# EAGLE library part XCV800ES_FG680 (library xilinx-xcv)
xcv800es_fg680 edit this description Auto generated by make-symbol-device-package-bsdl.ulp Rev. 26 Source: xcv800es_fg680.bsd
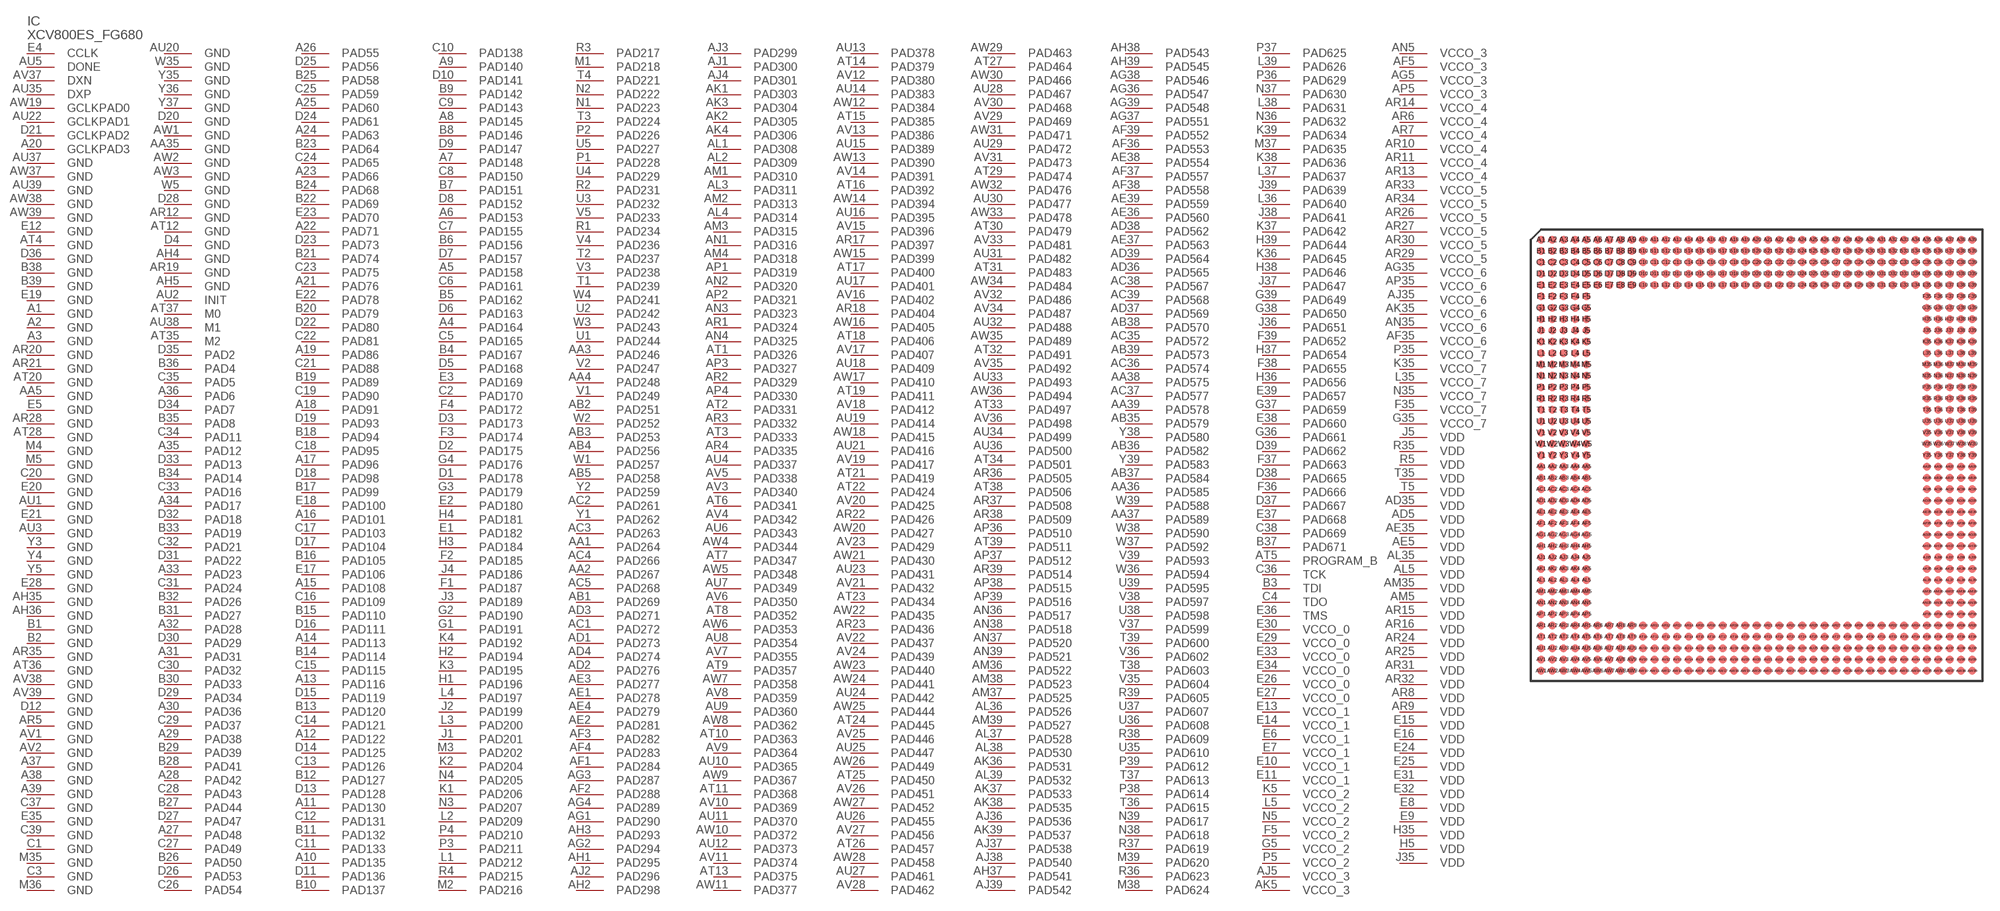
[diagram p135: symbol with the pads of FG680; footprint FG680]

Designator prefix IC

## XCV800ES_FG680 (OC_FARNELL: unknown; OC_NEWARK: unknown)  [FG680]
A1  GND  pwr
A2  GND  pwr
A3  GND  pwr
A4  PAD164
A5  PAD158
A6  PAD153
A7  PAD148
A8  PAD145
A9  PAD140
A10  PAD135
A11  PAD130
A12  PAD122
A13  PAD116
A14  PAD113
A15  PAD108
A16  PAD101
A17  PAD96
A18  PAD91
A19  PAD86
A20  GCLKPAD3  in
A21  PAD76
A22  PAD71
A23  PAD66
A24  PAD63
A25  PAD60
A26  PAD55
A27  PAD48
A28  PAD42
A29  PAD38
A30  PAD36
A31  PAD31
A32  PAD28
A33  PAD23
A34  PAD17
A35  PAD12
A36  PAD6
A37  GND  pwr
A38  GND  pwr
A39  GND  pwr
AA1  PAD264
AA2  PAD267
AA3  PAD246
AA4  PAD248
AA5  GND  pwr
AA35  GND  pwr
AA36  PAD585
AA37  PAD589
AA38  PAD575
AA39  PAD578
AB1  PAD269
AB2  PAD251
AB3  PAD253
AB4  PAD256
AB5  PAD258
AB35  PAD579
AB36  PAD582
AB37  PAD584
AB38  PAD570
AB39  PAD573
AC1  PAD272
AC2  PAD261
AC3  PAD263
AC4  PAD266
AC5  PAD268
AC35  PAD572
AC36  PAD574
AC37  PAD577
AC38  PAD567
AC39  PAD568
AD1  PAD273
AD2  PAD276
AD3  PAD271
AD4  PAD274
AD5  VDD  pwr
AD35  VDD  pwr
AD36  PAD565
AD37  PAD569
AD38  PAD562
AD39  PAD564
AE1  PAD278
AE2  PAD281
AE3  PAD277
AE4  PAD279
AE5  VDD  pwr
AE35  VDD  pwr
AE36  PAD560
AE37  PAD563
AE38  PAD554
AE39  PAD559
AF1  PAD284
AF2  PAD288
AF3  PAD282
AF4  PAD283
AF5  VCCO_3  pwr
AF35  VCCO_6  pwr
AF36  PAD553
AF37  PAD557
AF38  PAD558
AF39  PAD552
AG1  PAD290
AG2  PAD294
AG3  PAD287
AG4  PAD289
AG5  VCCO_3  pwr
AG35  VCCO_6  pwr
AG36  PAD547
AG37  PAD551
AG38  PAD546
AG39  PAD548
AH1  PAD295
AH2  PAD298
AH3  PAD293
AH4  GND  pwr
AH5  GND  pwr
AH35  GND  pwr
AH36  GND  pwr
AH37  PAD541
AH38  PAD543
AH39  PAD545
AJ1  PAD300
AJ2  PAD296
AJ3  PAD299
AJ4  PAD301
AJ5  VCCO_3  pwr
AJ35  VCCO_6  pwr
AJ36  PAD536
AJ37  PAD538
AJ38  PAD540
AJ39  PAD542
AK1  PAD303
AK2  PAD305
AK3  PAD304
AK4  PAD306
AK5  VCCO_3  pwr
AK35  VCCO_6  pwr
AK36  PAD531
AK37  PAD533
AK38  PAD535
AK39  PAD537
AL1  PAD308
AL2  PAD309
AL3  PAD311
AL4  PAD314
AL5  VDD  pwr
AL35  VDD  pwr
AL36  PAD526
AL37  PAD528
AL38  PAD530
AL39  PAD532
AM1  PAD310
AM2  PAD313
AM3  PAD315
AM4  PAD318
AM5  VDD  pwr
AM35  VDD  pwr
AM36  PAD522
AM37  PAD525
AM38  PAD523
AM39  PAD527
AN1  PAD316
AN2  PAD320
AN3  PAD323
AN4  PAD325
AN5  VCCO_3  pwr
AN35  VCCO_6  pwr
AN36  PAD517
AN37  PAD520
AN38  PAD518
AN39  PAD521
AP1  PAD319
AP2  PAD321
AP3  PAD327
AP4  PAD330
AP5  VCCO_3  pwr
AP35  VCCO_6  pwr
AP36  PAD510
AP37  PAD512
AP38  PAD515
AP39  PAD516
AR1  PAD324
AR2  PAD329
AR3  PAD332
AR4  PAD335
AR5  GND  pwr
AR6  VCCO_4  pwr
AR7  VCCO_4  pwr
AR8  VDD  pwr
AR9  VDD  pwr
AR10  VCCO_4  pwr
AR11  VCCO_4  pwr
AR12  GND  pwr
AR13  VCCO_4  pwr
AR14  VCCO_4  pwr
AR15  VDD  pwr
AR16  VDD  pwr
AR17  PAD397
AR18  PAD404
AR19  GND  pwr
AR20  GND  pwr
AR21  GND  pwr
AR22  PAD426
AR23  PAD436
AR24  VDD  pwr
AR25  VDD  pwr
AR26  VCCO_5  pwr
AR27  VCCO_5  pwr
AR28  GND  pwr
AR29  VCCO_5  pwr
AR30  VCCO_5  pwr
AR31  VDD  pwr
AR32  VDD  pwr
AR33  VCCO_5  pwr
AR34  VCCO_5  pwr
AR35  GND  pwr
AR36  PAD505
AR37  PAD508
AR38  PAD509
AR39  PAD514
AT1  PAD326
AT2  PAD331
AT3  PAD333
AT4  GND  pwr
AT5  PROGRAM_B  in
AT6  PAD341
AT7  PAD347
AT8  PAD352
AT9  PAD357
AT10  PAD363
AT11  PAD368
AT12  GND  pwr
AT13  PAD375
AT14  PAD379
AT15  PAD385
AT16  PAD392
AT17  PAD400
AT18  PAD406
AT19  PAD411
AT20  GND  pwr
AT21  PAD419
AT22  PAD424
AT23  PAD434
AT24  PAD445
AT25  PAD450
AT26  PAD457
AT27  PAD464
AT28  GND  pwr
AT29  PAD474
AT30  PAD479
AT31  PAD483
AT32  PAD491
AT33  PAD497
AT34  PAD501
AT35  M2  in
AT36  GND  pwr
AT37  M0  in
AT38  PAD506
AT39  PAD511
AU1  GND  pwr
AU2  INIT
AU3  GND  pwr
AU4  PAD337
AU5  DONE
AU6  PAD343
AU7  PAD349
AU8  PAD354
AU9  PAD360
AU10  PAD365
AU11  PAD370
AU12  PAD373
AU13  PAD378
AU14  PAD383
AU15  PAD389
AU16  PAD395
AU17  PAD401
AU18  PAD409
AU19  PAD414
AU20  GND  pwr
AU21  PAD416
AU22  GCLKPAD1  in
AU23  PAD431
AU24  PAD442
AU25  PAD447
AU26  PAD455
AU27  PAD461
AU28  PAD467
AU29  PAD472
AU30  PAD477
AU31  PAD482
AU32  PAD488
AU33  PAD493
AU34  PAD499
AU35  DXP  pas
AU36  PAD500
AU37  GND  pwr
AU38  M1  in
AU39  GND  pwr
AV1  GND  pwr
AV2  GND  pwr
AV3  PAD340
AV4  PAD342
AV5  PAD338
AV6  PAD350
AV7  PAD355
AV8  PAD359
AV9  PAD364
AV10  PAD369
AV11  PAD374
AV12  PAD380
AV13  PAD386
AV14  PAD391
AV15  PAD396
AV16  PAD402
AV17  PAD407
AV18  PAD412
AV19  PAD417
AV20  PAD425
AV21  PAD432
AV22  PAD437
AV23  PAD429
AV24  PAD439
AV25  PAD446
AV26  PAD451
AV27  PAD456
AV28  PAD462
AV29  PAD469
AV30  PAD468
AV31  PAD473
AV32  PAD486
AV33  PAD481
AV34  PAD487
AV35  PAD492
AV36  PAD498
AV37  DXN  pas
AV38  GND  pwr
AV39  GND  pwr
AW1  GND  pwr
AW2  GND  pwr
AW3  GND  pwr
AW4  PAD344
AW5  PAD348
AW6  PAD353
AW7  PAD358
AW8  PAD362
AW9  PAD367
AW10  PAD372
AW11  PAD377
AW12  PAD384
AW13  PAD390
AW14  PAD394
AW15  PAD399
AW16  PAD405
AW17  PAD410
AW18  PAD415
AW19  GCLKPAD0  in
AW20  PAD427
AW21  PAD430
AW22  PAD435
AW23  PAD440
AW24  PAD441
AW25  PAD444
AW26  PAD449
AW27  PAD452
AW28  PAD458
AW29  PAD463
AW30  PAD466
AW31  PAD471
AW32  PAD476
AW33  PAD478
AW34  PAD484
AW35  PAD489
AW36  PAD494
AW37  GND  pwr
AW38  GND  pwr
AW39  GND  pwr
B1  GND  pwr
B2  GND  pwr
B3  TDI  in
B4  PAD167
B5  PAD162
B6  PAD156
B7  PAD151
B8  PAD146
B9  PAD142
B10  PAD137
B11  PAD132
B12  PAD127
B13  PAD120
B14  PAD114
B15  PAD110
B16  PAD105
B17  PAD99
B18  PAD94
B19  PAD89
B20  PAD79
B21  PAD74
B22  PAD69
B23  PAD64
B24  PAD68
B25  PAD58
B26  PAD50
B27  PAD44
B28  PAD41
B29  PAD39
B30  PAD33
B31  PAD27
B32  PAD26
B33  PAD19
B34  PAD14
B35  PAD8
B36  PAD4
B37  PAD671
B38  GND  pwr
B39  GND  pwr
C1  GND  pwr
C2  PAD170
C3  GND  pwr
C4  TDO  out
C5  PAD165
C6  PAD161
C7  PAD155
C8  PAD150
C9  PAD143
C10  PAD138
C11  PAD133
C12  PAD131
C13  PAD126
C14  PAD121
C15  PAD115
C16  PAD109
C17  PAD103
C18  PAD95
C19  PAD90
C20  GND  pwr
C21  PAD88
C22  PAD81
C23  PAD75
C24  PAD65
C25  PAD59
C26  PAD54
C27  PAD49
C28  PAD43
C29  PAD37
C30  PAD32
C31  PAD24
C32  PAD21
C33  PAD16
C34  PAD11
C35  PAD5
C36  TCK  in
C37  GND  pwr
C38  PAD669
C39  GND  pwr
D1  PAD178
D2  PAD175
D3  PAD173
D4  GND  pwr
D5  PAD168
D6  PAD163
D7  PAD157
D8  PAD152
D9  PAD147
D10  PAD141
D11  PAD136
D12  GND  pwr
D13  PAD128
D14  PAD125
D15  PAD119
D16  PAD111
D17  PAD104
D18  PAD98
D19  PAD93
D20  GND  pwr
D21  GCLKPAD2  in
D22  PAD80
D23  PAD73
D24  PAD61
D25  PAD56
D26  PAD53
D27  PAD47
D28  GND  pwr
D29  PAD34
D30  PAD29
D31  PAD22
D32  PAD18
D33  PAD13
D34  PAD7
D35  PAD2
D36  GND  pwr
D37  PAD667
D38  PAD665
D39  PAD662
E1  PAD182
E2  PAD180
E3  PAD169
E4  CCLK
E5  GND  pwr
E6  VCCO_1  pwr
E7  VCCO_1  pwr
E8  VDD  pwr
E9  VDD  pwr
E10  VCCO_1  pwr
E11  VCCO_1  pwr
E12  GND  pwr
E13  VCCO_1  pwr
E14  VCCO_1  pwr
E15  VDD  pwr
E16  VDD  pwr
E17  PAD106
E18  PAD100
E19  GND  pwr
E20  GND  pwr
E21  GND  pwr
E22  PAD78
E23  PAD70
E24  VDD  pwr
E25  VDD  pwr
E26  VCCO_0  pwr
E27  VCCO_0  pwr
E28  GND  pwr
E29  VCCO_0  pwr
E30  VCCO_0  pwr
E31  VDD  pwr
E32  VDD  pwr
E33  VCCO_0  pwr
E34  VCCO_0  pwr
E35  GND  pwr
E36  TMS  in
E37  PAD668
E38  PAD660
E39  PAD657
F1  PAD187
F2  PAD185
F3  PAD174
F4  PAD172
F5  VCCO_2  pwr
F35  VCCO_7  pwr
F36  PAD666
F37  PAD663
F38  PAD655
F39  PAD652
G1  PAD191
G2  PAD190
G3  PAD179
G4  PAD176
G5  VCCO_2  pwr
G35  VCCO_7  pwr
G36  PAD661
G37  PAD659
G38  PAD650
G39  PAD649
H1  PAD196
H2  PAD194
H3  PAD184
H4  PAD181
H5  VDD  pwr
H35  VDD  pwr
H36  PAD656
H37  PAD654
H38  PAD646
H39  PAD644
J1  PAD201
J2  PAD199
J3  PAD189
J4  PAD186
J5  VDD  pwr
J35  VDD  pwr
J36  PAD651
J37  PAD647
J38  PAD641
J39  PAD639
K1  PAD206
K2  PAD204
K3  PAD195
K4  PAD192
K5  VCCO_2  pwr
K35  VCCO_7  pwr
K36  PAD645
K37  PAD642
K38  PAD636
K39  PAD634
L1  PAD212
L2  PAD209
L3  PAD200
L4  PAD197
L5  VCCO_2  pwr
L35  VCCO_7  pwr
L36  PAD640
L37  PAD637
L38  PAD631
L39  PAD626
M1  PAD218
M2  PAD216
M3  PAD202
M4  GND  pwr
M5  GND  pwr
M35  GND  pwr
M36  GND  pwr
M37  PAD635
M38  PAD624
M39  PAD620
N1  PAD223
N2  PAD222
N3  PAD207
N4  PAD205
N5  VCCO_2  pwr
N35  VCCO_7  pwr
N36  PAD632
N37  PAD630
N38  PAD618
N39  PAD617
P1  PAD228
P2  PAD226
P3  PAD211
P4  PAD210
P5  VCCO_2  pwr
P35  VCCO_7  pwr
P36  PAD629
P37  PAD625
P38  PAD614
P39  PAD612
R1  PAD234
R2  PAD231
R3  PAD217
R4  PAD215
R5  VDD  pwr
R35  VDD  pwr
R36  PAD623
R37  PAD619
R38  PAD609
R39  PAD605
T1  PAD239
T2  PAD237
T3  PAD224
T4  PAD221
T5  VDD  pwr
T35  VDD  pwr
T36  PAD615
T37  PAD613
T38  PAD603
T39  PAD600
U1  PAD244
U2  PAD242
U3  PAD232
U4  PAD229
U5  PAD227
U35  PAD610
U36  PAD608
U37  PAD607
U38  PAD598
U39  PAD595
V1  PAD249
V2  PAD247
V3  PAD238
V4  PAD236
V5  PAD233
V35  PAD604
V36  PAD602
V37  PAD599
V38  PAD597
V39  PAD593
W1  PAD257
W2  PAD252
W3  PAD243
W4  PAD241
W5  GND  pwr
W35  GND  pwr
W36  PAD594
W37  PAD592
W38  PAD590
W39  PAD588
Y1  PAD262
Y2  PAD259
Y3  GND  pwr
Y4  GND  pwr
Y5  GND  pwr
Y35  GND  pwr
Y36  GND  pwr
Y37  GND  pwr
Y38  PAD580
Y39  PAD583

## Footprint FG680 (pad centres in mm)
xcv1000_fg680_1532 edit this description Auto generated by make-symbol-device-package-bsdl.ulp Rev. 26 Source: xcv1000_fg680_1532.bsd
smd 0.7 x 0.7: A1 -19,19; A2 -18,19; A3 -17,19; A4 -16,19; A5 -15,19; A6 -14,19; A7 -13,19; A8 -12,19; A9 -11,19; A10 -10,19; A11 -9,19; A12 -8,19; A13 -7,19; A14 -6,19; A15 -5,19; A16 -4,19; A17 -3,19; A18 -2,19; A19 -1,19; A20 0,19; A21 1,19; A22 2,19; A23 3,19; A24 4,19; A25 5,19; A26 6,19; A27 7,19; A28 8,19; A29 9,19; A30 10,19; A31 11,19; A32 12,19; A33 13,19; A34 14,19; A35 15,19; A36 16,19; A37 17,19; A38 18,19; A39 19,19; AA1 -19,-1; AA2 -18,-1; AA3 -17,-1; AA4 -16,-1; AA5 -15,-1; AA35 15,-1; AA36 16,-1; AA37 17,-1; AA38 18,-1; AA39 19,-1; AB1 -19,-2; AB2 -18,-2; AB3 -17,-2; AB4 -16,-2; AB5 -15,-2; AB35 15,-2; AB36 16,-2; AB37 17,-2; AB38 18,-2; AB39 19,-2; AC1 -19,-3; AC2 -18,-3; AC3 -17,-3; AC4 -16,-3; AC5 -15,-3; AC35 15,-3; AC36 16,-3; AC37 17,-3; AC38 18,-3; AC39 19,-3; AD1 -19,-4; AD2 -18,-4; AD3 -17,-4; AD4 -16,-4; AD5 -15,-4; AD35 15,-4; AD36 16,-4; AD37 17,-4; AD38 18,-4; AD39 19,-4; AE1 -19,-5; AE2 -18,-5; AE3 -17,-5; AE4 -16,-5; AE5 -15,-5; AE35 15,-5; AE36 16,-5; AE37 17,-5; AE38 18,-5; AE39 19,-5; AF1 -19,-6; AF2 -18,-6; AF3 -17,-6; AF4 -16,-6; AF5 -15,-6; AF35 15,-6; AF36 16,-6; AF37 17,-6; AF38 18,-6; AF39 19,-6; AG1 -19,-7; AG2 -18,-7; AG3 -17,-7; AG4 -16,-7; AG5 -15,-7; AG35 15,-7; AG36 16,-7; AG37 17,-7; AG38 18,-7; AG39 19,-7; AH1 -19,-8; AH2 -18,-8; AH3 -17,-8; AH4 -16,-8; AH5 -15,-8; AH35 15,-8; AH36 16,-8; AH37 17,-8; AH38 18,-8; AH39 19,-8; AJ1 -19,-9; AJ2 -18,-9; AJ3 -17,-9; AJ4 -16,-9; AJ5 -15,-9; AJ35 15,-9; AJ36 16,-9; AJ37 17,-9; AJ38 18,-9; AJ39 19,-9; AK1 -19,-10; AK2 -18,-10; AK3 -17,-10; AK4 -16,-10; AK5 -15,-10; AK35 15,-10; AK36 16,-10; AK37 17,-10; AK38 18,-10; AK39 19,-10; AL1 -19,-11; AL2 -18,-11; AL3 -17,-11; AL4 -16,-11; AL5 -15,-11; AL35 15,-11; AL36 16,-11; AL37 17,-11; AL38 18,-11; AL39 19,-11; AM1 -19,-12; AM2 -18,-12; AM3 -17,-12; AM4 -16,-12; AM5 -15,-12; AM35 15,-12; AM36 16,-12; AM37 17,-12; AM38 18,-12; AM39 19,-12; AN1 -19,-13; AN2 -18,-13; AN3 -17,-13; AN4 -16,-13; AN5 -15,-13; AN35 15,-13; AN36 16,-13; AN37 17,-13; AN38 18,-13; AN39 19,-13; AP1 -19,-14; AP2 -18,-14; AP3 -17,-14; AP4 -16,-14; AP5 -15,-14; AP35 15,-14; AP36 16,-14; AP37 17,-14; AP38 18,-14; AP39 19,-14; AR1 -19,-15; AR2 -18,-15; AR3 -17,-15; AR4 -16,-15; AR5 -15,-15; AR6 -14,-15; AR7 -13,-15; AR8 -12,-15; AR9 -11,-15; AR10 -10,-15; AR11 -9,-15; AR12 -8,-15; AR13 -7,-15; AR14 -6,-15; AR15 -5,-15; AR16 -4,-15; AR17 -3,-15; AR18 -2,-15; AR19 -1,-15; AR20 0,-15; AR21 1,-15; AR22 2,-15; AR23 3,-15; AR24 4,-15; AR25 5,-15; AR26 6,-15; AR27 7,-15; AR28 8,-15; AR29 9,-15; AR30 10,-15; AR31 11,-15; AR32 12,-15; AR33 13,-15; AR34 14,-15; AR35 15,-15; AR36 16,-15; AR37 17,-15; AR38 18,-15; AR39 19,-15; AT1 -19,-16; AT2 -18,-16; AT3 -17,-16; AT4 -16,-16; AT5 -15,-16; AT6 -14,-16; AT7 -13,-16; AT8 -12,-16; AT9 -11,-16; AT10 -10,-16; AT11 -9,-16; AT12 -8,-16; AT13 -7,-16; AT14 -6,-16; AT15 -5,-16; AT16 -4,-16; AT17 -3,-16; AT18 -2,-16; AT19 -1,-16; AT20 0,-16; AT21 1,-16; AT22 2,-16; AT23 3,-16; AT24 4,-16; AT25 5,-16; AT26 6,-16; AT27 7,-16; AT28 8,-16; AT29 9,-16; AT30 10,-16; AT31 11,-16; AT32 12,-16; AT33 13,-16; AT34 14,-16; AT35 15,-16; AT36 16,-16; AT37 17,-16; AT38 18,-16; AT39 19,-16; AU1 -19,-17; AU2 -18,-17; AU3 -17,-17; AU4 -16,-17; AU5 -15,-17; AU6 -14,-17; AU7 -13,-17; AU8 -12,-17; AU9 -11,-17; AU10 -10,-17; AU11 -9,-17; AU12 -8,-17; AU13 -7,-17; AU14 -6,-17; AU15 -5,-17; AU16 -4,-17; AU17 -3,-17; AU18 -2,-17; AU19 -1,-17; AU20 0,-17; AU21 1,-17; AU22 2,-17; AU23 3,-17; AU24 4,-17; AU25 5,-17; AU26 6,-17; AU27 7,-17; AU28 8,-17; AU29 9,-17; AU30 10,-17; AU31 11,-17; AU32 12,-17; AU33 13,-17; AU34 14,-17; AU35 15,-17; AU36 16,-17; AU37 17,-17; AU38 18,-17; AU39 19,-17; AV1 -19,-18; AV2 -18,-18; AV3 -17,-18; AV4 -16,-18; AV5 -15,-18; AV6 -14,-18; AV7 -13,-18; AV8 -12,-18; AV9 -11,-18; AV10 -10,-18; AV11 -9,-18; AV12 -8,-18; AV13 -7,-18; AV14 -6,-18; AV15 -5,-18; AV16 -4,-18; AV17 -3,-18; AV18 -2,-18; AV19 -1,-18; AV20 0,-18; AV21 1,-18; AV22 2,-18; AV23 3,-18; AV24 4,-18; AV25 5,-18; AV26 6,-18; AV27 7,-18; AV28 8,-18; AV29 9,-18; AV30 10,-18; AV31 11,-18; AV32 12,-18; AV33 13,-18; AV34 14,-18; AV35 15,-18; AV36 16,-18; AV37 17,-18; AV38 18,-18; AV39 19,-18; AW1 -19,-19; AW2 -18,-19; AW3 -17,-19; AW4 -16,-19; AW5 -15,-19; AW6 -14,-19; AW7 -13,-19; AW8 -12,-19; AW9 -11,-19; AW10 -10,-19; AW11 -9,-19; AW12 -8,-19; AW13 -7,-19; AW14 -6,-19; AW15 -5,-19; AW16 -4,-19; AW17 -3,-19; AW18 -2,-19; AW19 -1,-19; AW20 0,-19; AW21 1,-19; AW22 2,-19; AW23 3,-19; AW24 4,-19; AW25 5,-19; AW26 6,-19; AW27 7,-19; AW28 8,-19; AW29 9,-19; AW30 10,-19; AW31 11,-19; AW32 12,-19; AW33 13,-19; AW34 14,-19; AW35 15,-19; AW36 16,-19; AW37 17,-19; AW38 18,-19; AW39 19,-19; B1 -19,18; B2 -18,18; B3 -17,18; B4 -16,18; B5 -15,18; B6 -14,18; B7 -13,18; B8 -12,18; B9 -11,18; B10 -10,18; B11 -9,18; B12 -8,18; B13 -7,18; B14 -6,18; B15 -5,18; B16 -4,18; B17 -3,18; B18 -2,18; B19 -1,18; B20 0,18; B21 1,18; B22 2,18; B23 3,18; B24 4,18; B25 5,18; B26 6,18; B27 7,18; B28 8,18; B29 9,18; B30 10,18; B31 11,18; B32 12,18; B33 13,18; B34 14,18; B35 15,18; B36 16,18; B37 17,18; B38 18,18; B39 19,18; C1 -19,17; C2 -18,17; C3 -17,17; C4 -16,17; C5 -15,17; C6 -14,17; C7 -13,17; C8 -12,17; C9 -11,17; C10 -10,17; C11 -9,17; C12 -8,17; C13 -7,17; C14 -6,17; C15 -5,17; C16 -4,17; C17 -3,17; C18 -2,17; C19 -1,17; C20 0,17; C21 1,17; C22 2,17; C23 3,17; C24 4,17; C25 5,17; C26 6,17; C27 7,17; C28 8,17; C29 9,17; C30 10,17; C31 11,17; C32 12,17; C33 13,17; C34 14,17; C35 15,17; C36 16,17; C37 17,17; C38 18,17; C39 19,17; D1 -19,16; D2 -18,16; D3 -17,16; D4 -16,16; D5 -15,16; D6 -14,16; D7 -13,16; D8 -12,16; D9 -11,16; D10 -10,16; D11 -9,16; D12 -8,16; D13 -7,16; D14 -6,16; D15 -5,16; D16 -4,16; D17 -3,16; D18 -2,16; D19 -1,16; D20 0,16; D21 1,16; D22 2,16; D23 3,16; D24 4,16; D25 5,16; D26 6,16; D27 7,16; D28 8,16; D29 9,16; D30 10,16; D31 11,16; D32 12,16; D33 13,16; D34 14,16; D35 15,16; D36 16,16; D37 17,16; D38 18,16; D39 19,16; E1 -19,15; E2 -18,15; E3 -17,15; E4 -16,15; E5 -15,15; E6 -14,15; E7 -13,15; E8 -12,15; E9 -11,15; E10 -10,15; E11 -9,15; E12 -8,15; E13 -7,15; E14 -6,15; E15 -5,15; E16 -4,15; E17 -3,15; E18 -2,15; E19 -1,15; E20 0,15; E21 1,15; E22 2,15; E23 3,15; E24 4,15; E25 5,15; E26 6,15; E27 7,15; E28 8,15; E29 9,15; E30 10,15; E31 11,15; E32 12,15; E33 13,15; E34 14,15; E35 15,15; E36 16,15; E37 17,15; E38 18,15; E39 19,15; F1 -19,14; F2 -18,14; F3 -17,14; F4 -16,14; F5 -15,14; F35 15,14; F36 16,14; F37 17,14; F38 18,14; F39 19,14; G1 -19,13; G2 -18,13; G3 -17,13; G4 -16,13; G5 -15,13; G35 15,13; G36 16,13; G37 17,13; G38 18,13; G39 19,13; H1 -19,12; H2 -18,12; H3 -17,12; H4 -16,12; H5 -15,12; H35 15,12; H36 16,12; H37 17,12; H38 18,12; H39 19,12; J1 -19,11; J2 -18,11; J3 -17,11; J4 -16,11; J5 -15,11; J35 15,11; J36 16,11; J37 17,11; J38 18,11; J39 19,11; K1 -19,10; K2 -18,10; K3 -17,10; K4 -16,10; K5 -15,10; K35 15,10; K36 16,10; K37 17,10; K38 18,10; K39 19,10; L1 -19,9; L2 -18,9; L3 -17,9; L4 -16,9; L5 -15,9; L35 15,9; L36 16,9; L37 17,9; L38 18,9; L39 19,9; M1 -19,8; M2 -18,8; M3 -17,8; M4 -16,8; M5 -15,8; M35 15,8; M36 16,8; M37 17,8; M38 18,8; M39 19,8; N1 -19,7; N2 -18,7; N3 -17,7; N4 -16,7; N5 -15,7; N35 15,7; N36 16,7; N37 17,7; N38 18,7; N39 19,7; P1 -19,6; P2 -18,6; P3 -17,6; P4 -16,6; P5 -15,6; P35 15,6; P36 16,6; P37 17,6; P38 18,6; P39 19,6; R1 -19,5; R2 -18,5; R3 -17,5; R4 -16,5; R5 -15,5; R35 15,5; R36 16,5; R37 17,5; R38 18,5; R39 19,5; T1 -19,4; T2 -18,4; T3 -17,4; T4 -16,4; T5 -15,4; T35 15,4; T36 16,4; T37 17,4; T38 18,4; T39 19,4; U1 -19,3; U2 -18,3; U3 -17,3; U4 -16,3; U5 -15,3; U35 15,3; U36 16,3; U37 17,3; U38 18,3; U39 19,3; V1 -19,2; V2 -18,2; V3 -17,2; V4 -16,2; V5 -15,2; V35 15,2; V36 16,2; V37 17,2; V38 18,2; V39 19,2; W1 -19,1; W2 -18,1; W3 -17,1; W4 -16,1; W5 -15,1; W35 15,1; W36 16,1; W37 17,1; W38 18,1; W39 19,1; Y1 -19,0; Y2 -18,0; Y3 -17,0; Y4 -16,0; Y5 -15,0; Y35 15,0; Y36 16,0; Y37 17,0; Y38 18,0; Y39 19,0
